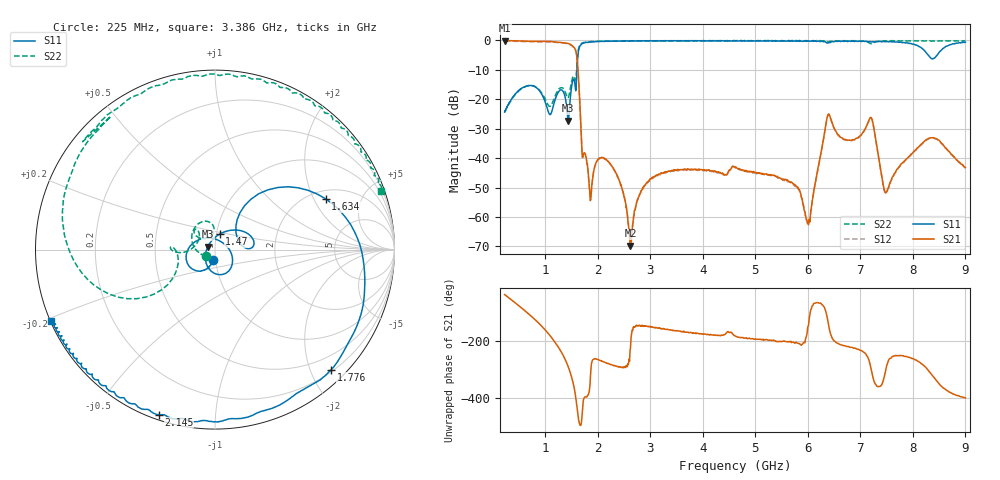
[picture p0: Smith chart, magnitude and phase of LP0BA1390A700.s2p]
!Agilent Technologies,E8358A,US41080443,A.07.50.56
!Agilent E8358A: A.07.50.56
!Date: Monday, May 09, 2016 11:49:38
!Correction: S11(Full 2 Port(1,2))
!S21(Full 2 Port(1,2))
!S12(Full 2 Port(1,2))
!S22(Full 2 Port(1,2))
!S2P File: Measurements: S11, S21, S12, S22:Log Frequency Sweep
# Hz S  dB  R 50
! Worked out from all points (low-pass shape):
!   1601 points, 225 MHz to 9 GHz, reference 50 ohm
!   highest |S21| = -0.01 dB at 226 MHz (marker M1); lowest = -69.7 dB at 2.622 GHz (marker M2)
!   |S21| within 3 dB of the highest: start of sweep to 1.571 GHz
!   lowest |S11| = -27.3 dB at 1.436 GHz (marker M3), VSWR 1.09, Z = 46.1 + j1.55 ohm
!   |S11| at or under -10 dB: start of sweep to 1.602 GHz
!   |S22| runs from -24.5 to 0.0 dB; largest |S21 - S12| = 0.021
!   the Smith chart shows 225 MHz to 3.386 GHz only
!   S11 on the Smith chart (normalised r, x): 225 MHz: 0.97, -0.12; 1.47 GHz: 1.04, +0.18; 1.634 GHz: 2.37, +2.49; 1.776 GHz: 0.23, -2.34; 2.145 GHz: 0.02, -0.72; 3.386 GHz: 0.00, -0.21
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2.25e8  -24.31 -98.9  -0.02 -32.7  -0.18 -32.6  -24.48 -146.0
2.260399e8  -24.26 -99.1  -0.01 -32.9  -0.18 -32.7  -24.44 -146.4
6.618889e8  -15.39 -144.6  -0.26 -98.6  -0.43 -98.4  -15.45 128.7
1.05937e9  -24.33 94.7  -0.33 -172.3  -0.50 -172.1  -22.08 107.1
1.436209e9  -27.30 157.2  -1.02 69.9  -1.19 70.1  -19.47 159.4
1.469706e9  -20.90 73.4  -1.23 52.0  -1.41 52.1  -17.02 -179.0
1.634142e9  -3.38 24.7  -13.32 -119.0  -13.47 -119.2  -2.73 -167.0
1.687749e9  -1.30 -14.5  -33.61 -129.5  -33.73 -129.9  -0.99 160.3
1.775563e9  -0.63 -45.9  -39.60 -37.7  -39.87 -37.5  -0.58 132.7
1.863645e9  -0.56 -73.6  -53.73 46.9  -53.90 48.7  -0.36 129.5
2.145071e9  -0.25 -108.8  -40.29 84.5  -40.41 84.9  -0.25 95.1
2.621523e9  -0.13 -136.6  -69.73 135.6  -69.92 134.0  -0.17 58.8
3.152512e9  -0.14 -152.3  -45.51 -151.9  -45.74 -151.7  -0.11 29.9
3.386075e9  -0.06 -156.5  -44.35 -158.8  -44.63 -158.8  -0.19 19.5
4.622431e9  -0.12 -175.7  -43.09 178.9  -43.43 178.8  -0.11 -15.5
6.081681e9  -0.20 156.2  -54.80 -72.6  -54.54 -74.1  -0.10 -36.3
6.427684e9  -0.68 152.5  -26.20 -170.2  -26.25 -170.5  -0.25 -39.6
7.179866e9  -0.37 134.1  -26.37 82.2  -26.64 82.8  -0.97 -53.1
7.553438e9  -0.41 124.4  -48.88 98.4  -49.14 96.6  -0.14 -55.6
8.283162e9  -4.78 21.7  -33.45 58.9  -33.65 59.4  -0.19 -68.6
8.535184e9  -3.41 -124.4  -34.71 1.6  -34.90 1.1  -0.16 -73.9
9e9  -0.59 171.9  -43.16 -41.4  -43.50 -42.1  -0.16 -81.5
